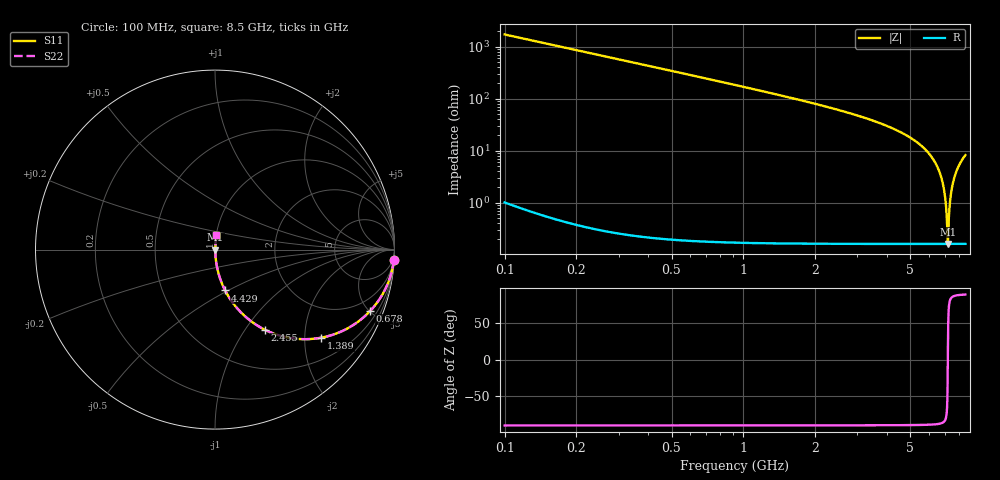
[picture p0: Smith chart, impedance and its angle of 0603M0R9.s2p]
! Created Wed Apr 18 12:03:55 2012
# hz S ma R 50
! 2 Port Network Data from SP1.SP block
! freq  magS11  angS11  magS21  angS21  magS12  angS12  magS22  angS22
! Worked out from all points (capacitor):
!   8401 points, 100 MHz to 8.5 GHz, reference 50 ohm
!   read as one part in series: C = 920 fF near 142 MHz
!   lowest |Z| = 160 mohm at 7.175 GHz (marker M1)
!   series resonance near 7.175 GHz, so ESL is about 530 pH
!   S11 on the Smith chart (normalised r, x): 100 MHz: 1, -35; 678 MHz: 1.00, -5.06; 1.389 GHz: 1.00, -2.40; 2.455 GHz: 1.00, -1.24; 4.429 GHz: 1.00, -0.48; 8.5 GHz: 1.00, +0.16
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1e8  0.9983 -3.3  0.05772 86.7  0.05772 86.7  0.9983 -3.3
3.21e8  0.9831 -10.5  0.1828 79.4  0.1828 79.4  0.9831 -10.5
6.78e8  0.9297 -21.6  0.3676 68.4  0.3676 68.4  0.9297 -21.6
1.389e9  0.7674 -39.8  0.6401 50.1  0.6401 50.1  0.7674 -39.8
1.5e9  0.7403 -42.2  0.6712 47.8  0.6712 47.8  0.7403 -42.2
2.455e9  0.5277 -58.0  0.8481 31.9  0.8481 31.9  0.5277 -58.0
2.9e9  0.4461 -63.3  0.8936 26.5  0.8936 26.5  0.4461 -63.3
4.3e9  0.2494 -75.2  0.9669 14.4  0.9669 14.4  0.2494 -75.2
4.429e9  0.2348 -76.0  0.9705 13.6  0.9705 13.6  0.2348 -76.0
5.7e9  0.1112 -82.8  0.9922 6.4  0.9922 6.4  0.1112 -82.8
6.297e9  0.063 -84.9  0.9964 3.6  0.9964 3.6  0.063 -84.9
6.704e9  0.0328 -85.3  0.9979 1.9  0.9979 1.9  0.0328 -85.3
6.959e9  0.01485 -83.0  0.9983 0.8  0.9983 0.8  0.01485 -83.0
7.041e9  0.009251 -79.5  0.9984 0.5  0.9984 0.5  0.009251 -79.5
7.1e9  0.005335 -72.3  0.9984 0.3  0.9984 0.3  0.005335 -72.3
7.148e9  0.002439 -48.9  0.9984 0.1  0.9984 0.1  0.002439 -48.9
7.175e9  0.001601 -0.8  0.9984 0.0  0.9984 0.0  0.001601 -0.8
7.2e9  0.002301 45.8  0.9984 -0.1  0.9984 -0.1  0.002301 45.8
7.324e9  0.01001 80.2  0.9984 -0.6  0.9984 -0.6  0.01001 80.2
7.533e9  0.02351 84.8  0.9981 -1.3  0.9981 -1.3  0.02351 84.8
7.918e9  0.04754 85.3  0.9973 -2.7  0.9973 -2.7  0.04754 85.3
8.5e9  0.08185 84.2  0.995 -4.7  0.995 -4.7  0.08185 84.2
